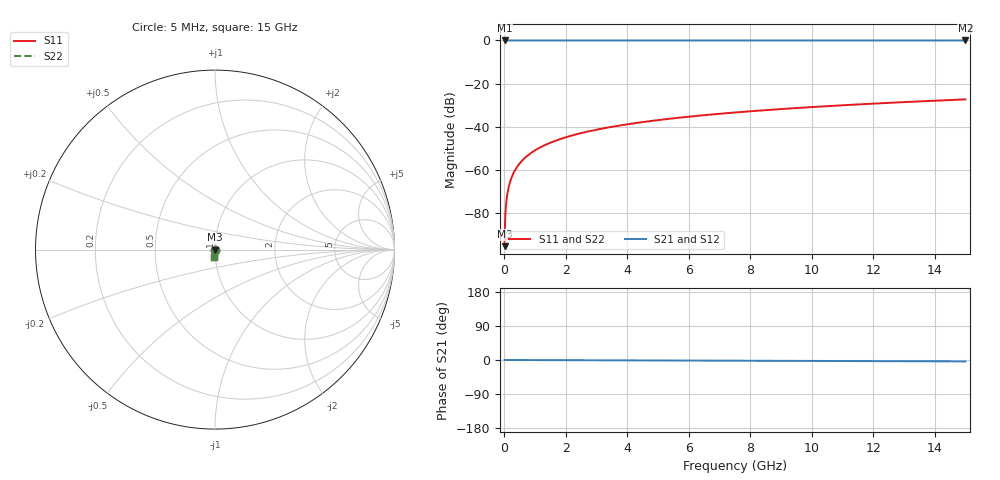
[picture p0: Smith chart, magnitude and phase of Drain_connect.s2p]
! Created Tue Jan 19 10:20:24 2021
# hz S ma R 50
! 2 Port Network Data from SP1.SP block
! freq  magS11  angS11  magS21  angS21  magS12  angS12  magS22  angS22
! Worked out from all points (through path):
!   3000 points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, 5 MHz to 15 GHz, reference 50 ohm
!   highest |S21| = 0.00 dB at 5 MHz (marker M1); lowest = 0.0 dB at 15 GHz (marker M2)
!   lowest |S11| = -95.5 dB at 5 MHz (marker M3), VSWR 1.00, Z = 50 - j0.00168 ohm
!   |S11| at or under -10 dB: start of sweep to end of sweep
!   |S22| runs from -95.5 to -27.4 dB; largest |S21 - S12| = 0
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5000000  1.682e-05 -91.2  1 -0.0  1 -0.0  1.682e-05 -91.2
5.5e7  0.000166 -94.8  1 -0.0  1 -0.0  0.000166 -94.8
1.2e8  0.0003464 -93.1  1 -0.0  1 -0.0  0.0003464 -93.1
1.45e8  0.0004163 -92.7  1 -0.0  1 -0.0  0.0004163 -92.7
1.85e8  0.0005286 -92.2  1 -0.0  1 -0.0  0.0005286 -92.2
2.35e8  0.0006694 -91.8  1 -0.1  1 -0.1  0.0006694 -91.8
3.1e8  0.0008812 -91.4  1 -0.1  1 -0.1  0.0008812 -91.4
3.95e8  0.001121 -91.1  1 -0.1  1 -0.1  0.001121 -91.1
4.95e8  0.001404 -90.9  1 -0.1  1 -0.1  0.001404 -90.9
6.15e8  0.001744 -90.8  1 -0.2  1 -0.2  0.001744 -90.8
7.65e8  0.002169 -90.7  1 -0.2  1 -0.2  0.002169 -90.7
9.35e8  0.002651 -90.7  1 -0.2  1 -0.2  0.002651 -90.7
1.345e9  0.003812 -90.6  1 -0.3  1 -0.3  0.003812 -90.6
1.865e9  0.005286 -90.7  1 -0.5  1 -0.5  0.005286 -90.7
2.505e9  0.0071 -90.7  1 -0.6  1 -0.6  0.0071 -90.7
3.61e9  0.01023 -91.0  0.9999 -0.9  0.9999 -0.9  0.01023 -91.0
5.005e9  0.0142 -91.3  0.9999 -1.2  0.9999 -1.2  0.0142 -91.3
6.17e9  0.01751 -91.5  0.9998 -1.5  0.9998 -1.5  0.01751 -91.5
7.505e9  0.02131 -91.9  0.9998 -1.8  0.9998 -1.8  0.02131 -91.9
1.0005e10  0.02846 -92.6  0.9995 -2.5  0.9995 -2.5  0.02846 -92.6
1.2505e10  0.03565 -93.3  0.9992 -3.1  0.9992 -3.1  0.03565 -93.3
1.5e10  0.04289 -94.2  0.9987 -3.7  0.9987 -3.7  0.04289 -94.2
